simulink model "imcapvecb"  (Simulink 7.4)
settings: Solver=ode45  StartTime=0  StopTime=2.5  MaxStep=5e-4  RelTol=1e-4

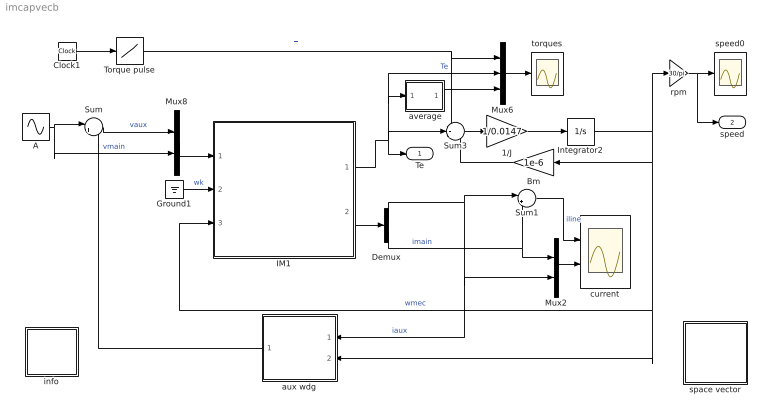
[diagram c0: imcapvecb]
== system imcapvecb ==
  " average" : Subsystem
  1/J : Gain  Gain=1/0.0147  ParameterDataType=sfix(16)  ParameterScaling=2^0  OutDataType=sfix(16)  OutScaling=2^0
  A : Sin  Amplitude=110*sqrt(2)  Bias=0  Frequency=2*pi*60  Phase=pi/2  Samples=10  SampleTime=0
  Bm : Gain  Gain=1e-6  ParameterDataType=sfix(16)  ParameterScaling=2^0  OutDataType=sfix(16)  OutScaling=2^0
  Clock1 : Clock
  Demux : Demux  Outputs=2
  Ground1 : Ground
  IM1 : Subsystem  mask(Inductionmachine){Rs=2.02, Rr=4.12, Lsl=8.54e-3, Lrl=3.13e-3, Lm=180e-3, wo=2*pi*60, p=4}
      mask prompts: Rs "Stator resistance [ohm]"; Rr "Rotor resistance [ohm]"; Lsl "Stator leakage inductance  [H]"; Lrl "Rotor leakage inductance [H]"; Lm "Magnetizing inductance [H]"; wo "Base frequency [rad/s]"; p "Number of poles"
      mask help: Space vector model of the induction machine in a general frame k. SI units
  Integrator2 : Integrator
  Mux2 : Mux  Inputs=2
  Mux6 : Mux  Inputs=3
  Mux8 : Mux  Inputs=2
  Sum : Sum  Inputs=|+-  OutDataType=sfix(16)  OutScaling=2^0
  Sum1 : Sum  Inputs=|++  OutDataType=sfix(16)  OutScaling=2^0
  Sum3 : Sum  Inputs=-+-  OutDataType=sfix(16)  OutScaling=2^0
  Torque pulse : Lookup  InputValues=[0 1 1 1.5 1.5 2]  Table=[0 0 3 3 1.3 1.3]  OutDataType=sfix(16)  OutScaling=2^0
  aux wdg : Subsystem  mask{Cstart=183e-6, p=4, Nsw=3/4}
      mask prompts: Cstart "Start capacitance [F]"; p "Number of poles"; Nsw "Speed when switch disconnects [pu]"
  current : Scope  NumInputPorts=2
  info : Subsystem
  rpm : Gain  Gain=30/pi  ParameterDataType=sfix(16)  ParameterScaling=2^0  OutDataType=sfix(16)  OutScaling=2^0
  space vector : Subsystem
  speed0 : Scope
  torques : Scope
  Te : Outport
  speed : Outport  Port=2
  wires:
  Sum1/1 -> current/1  "iline"
  Mux2/1 -> current/2
  Mux8/1 -> IM1/1(vs)
  Sum/1 -> Mux8/1  "vaux"
  A/1 -> Sum/1, Mux8/2  "vmain"
  IM1/2(is) -> Demux/1
  Demux/1 -> Sum1/1, aux wdg/1(ias), Mux2/2  "iaux"
  Demux/2 -> Sum1/2, Mux2/1  "imain"
  1/J/1 -> Integrator2/1
  Mux6/1 -> torques/1
  Bm/1 -> Sum3/3
  Integrator2/1 -> Bm/1, aux wdg/2(wmec), IM1/3(wmec), rpm/1  "wmec"
  rpm/1 -> speed/1, speed0/1
  IM1/1(Te) -> Sum3/2, Te/1, Mux6/2, " average"/1(sig)  "Te"
  aux wdg/1(vaux) -> Sum/2
  Sum3/1 -> 1/J/1
  Clock1/1 -> Torque pulse/1
  Torque pulse/1 -> Mux6/1, Sum3/1  "Tl"
  Ground1/1 -> IM1/2(wk)  "wk"
  " average"/1(ave) -> Mux6/3

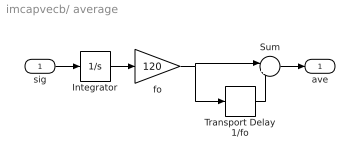
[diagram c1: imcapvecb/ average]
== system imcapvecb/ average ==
  sig : Inport  OutDataType=sfix(16)  OutScaling=2^0
  Integrator : Integrator
  Sum : Sum  Inputs=|+-  OutDataType=sfix(16)  OutScaling=2^0
  Transport Delay 1/fo : TransportDelay  DelayTime=1/120
  fo : Gain  Gain=120  ParameterDataType=sfix(16)  ParameterScaling=2^0  OutDataType=sfix(16)  OutScaling=2^0
  ave : Outport
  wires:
  Sum/1 -> ave/1
  Transport Delay 1/fo/1 -> Sum/2
  sig/1 -> Integrator/1
  fo/1 -> Transport Delay 1/fo/1, Sum/1
  Integrator/1 -> fo/1

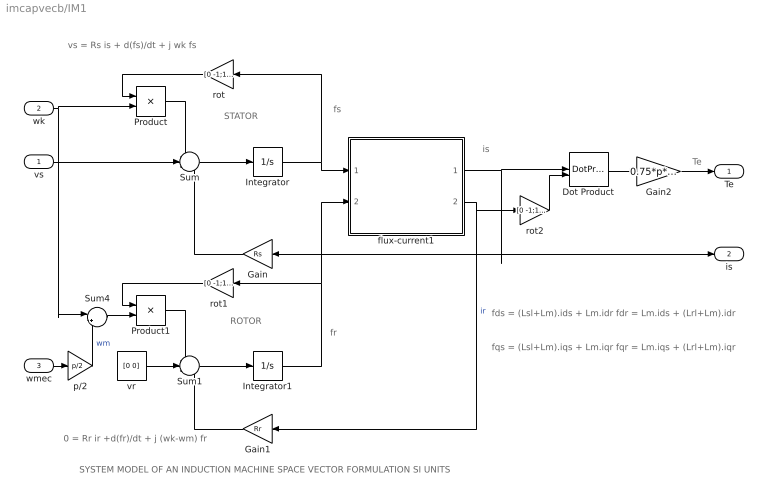
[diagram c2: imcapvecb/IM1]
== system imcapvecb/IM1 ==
  note: ROTOR
  note: STATOR
  note: fs
  note: is
  note: Te
  note: SYSTEM MODEL OF AN INDUCTION MACHINE SPACE VECTOR FORMULATION SI UNITS
  note: vs = Rs is + d(fs)/dt + j wk fs
  note: 0 = Rr ir +d(fr)/dt + j (wk-wm) fr
  note: fds = (Lsl+Lm).ids + Lm.idr fdr = Lm.ids + (Lrl+Lm).idr
  note: fqs = (Lsl+Lm).iqs + Lm.iqr fqr = Lm.iqs + (Lrl+Lm).iqr
  note: fr
  vs : Inport  OutDataType=sfix(16)  OutScaling=2^0
  wk : Inport  Port=2  OutDataType=sfix(16)  OutScaling=2^0
  wmec : Inport  Port=3  OutDataType=sfix(16)  OutScaling=2^0
  Dot Product : DotProduct  OutDataType=fixdt(1, 16)  OutScaling=2^-10
  Gain : Gain  Gain=Rs  ParameterDataType=sfix(16)  ParameterScaling=2^0  OutDataType=sfix(16)  OutScaling=2^0
  Gain1 : Gain  Gain=Rr  ParameterDataType=sfix(16)  ParameterScaling=2^0  OutDataType=sfix(16)  OutScaling=2^0
  Gain2 : Gain  Gain=0.75*p*Lm  ParameterDataType=sfix(16)  ParameterScaling=2^0  OutDataType=sfix(16)  OutScaling=2^0
  Integrator : Integrator  InitialCondition=[0 0]
  Integrator1 : Integrator  InitialCondition=[0 0]
  Product : Product  OutDataType=sfix(16)  OutScaling=2^0
  Product1 : Product  OutDataType=sfix(16)  OutScaling=2^0
  Sum : Sum  Inputs=-+-  OutDataType=sfix(16)  OutScaling=2^0
  Sum1 : Sum  Inputs=-+-  OutDataType=sfix(16)  OutScaling=2^0
  Sum4 : Sum  Inputs=|+-  OutDataType=sfix(16)  OutScaling=2^0
  flux-current1 : Subsystem
  p/2 : Gain  Gain=p/2  ParameterDataType=sfix(16)  ParameterScaling=2^0  OutDataType=sfix(16)  OutScaling=2^0
  rot : Gain  Gain=[0 -1;1 0]  Multiplication=Matrix(K*u)  ParameterDataType=sfix(16)  ParameterScaling=2^0  OutDataType=sfix(16)  OutScaling=2^0
  rot1 : Gain  Gain=[0 -1;1 0]  Multiplication=Matrix(K*u)  ParameterDataType=sfix(16)  ParameterScaling=2^0  OutDataType=sfix(16)  OutScaling=2^0
  rot2 : Gain  Gain=[0 -1;1 0]  Multiplication=Matrix(K*u)  ParameterDataType=sfix(16)  ParameterScaling=2^0  OutDataType=sfix(16)  OutScaling=2^0
  vr : Constant  Value=[0 0]  OutDataType=sfix(16)  OutScaling=2^0
  Te : Outport
  is : Outport  Port=2
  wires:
  Gain/1 -> Sum/3
  vr/1 -> Sum1/2
  Gain1/1 -> Sum1/3
  Integrator/1 -> flux-current1/1(fs), rot/1
  Integrator1/1 -> rot1/1, flux-current1/2(fr)
  Product1/1 -> Sum1/1
  rot1/1 -> Product1/1
  Product/1 -> Sum/1
  rot/1 -> Product/1
  Sum4/1 -> Product1/2
  vs/1 -> Sum/2
  wk/1 -> Product/2, Sum4/1
  Sum1/1 -> Integrator1/1
  Sum/1 -> Integrator/1
  flux-current1/1(is) -> Gain/1, is/1, Dot Product/1
  Dot Product/1 -> Gain2/1
  Gain2/1 -> Te/1
  wmec/1 -> p/2/1
  p/2/1 -> Sum4/2  "wm"
  rot2/1 -> Dot Product/2
  flux-current1/2(ir) -> Gain1/1, rot2/1  "ir"

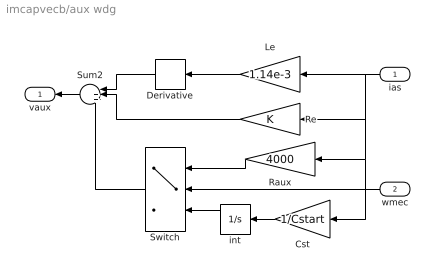
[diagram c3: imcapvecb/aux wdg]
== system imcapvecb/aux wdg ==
  ias : Inport  OutDataType=sfix(16)  OutScaling=2^0
  wmec : Inport  Port=2  OutDataType=sfix(16)  OutScaling=2^0
  Cst : Gain  Gain=1/Cstart  ParameterDataType=sfix(16)  ParameterScaling=2^0  OutDataType=sfix(16)  OutScaling=2^0
  Derivative : Derivative
  Le : Gain  Gain=1.14e-3  ParameterDataType=sfix(16)  ParameterScaling=2^0  OutDataType=sfix(16)  OutScaling=2^0
  Raux : Gain  Gain=4000  ParameterDataType=sfix(16)  ParameterScaling=2^0  OutDataType=sfix(16)  OutScaling=2^0
  Re : Gain  ParameterDataType=sfix(16)  ParameterScaling=2^0  OutDataType=sfix(16)  OutScaling=2^0
  Sum2 : Sum  Inputs=|+++  OutDataType=sfix(16)  OutScaling=2^0
  Switch : Switch  Threshold=Nsw*377*2/p
  int : Integrator
  vaux : Outport
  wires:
  Le/1 -> Derivative/1
  Derivative/1 -> Sum2/1
  Re/1 -> Sum2/2
  Cst/1 -> int/1
  Raux/1 -> Switch/1
  Switch/1 -> Sum2/3
  Sum2/1 -> vaux/1
  wmec/1 -> Switch/2
  ias/1 -> Cst/1, Raux/1, Re/1, Le/1
  int/1 -> Switch/3

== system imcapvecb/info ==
  note: This demo simulates the starting characteristics of a capacitor-start single-phase induction motor

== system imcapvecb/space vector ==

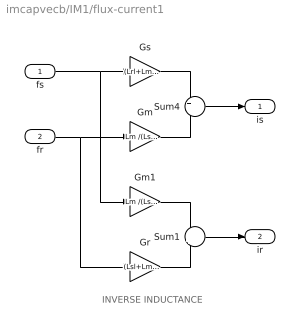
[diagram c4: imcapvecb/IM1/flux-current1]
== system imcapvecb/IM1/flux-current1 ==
  note: INVERSE INDUCTANCE
  fs : Inport  OutDataType=sfix(16)  OutScaling=2^0
  fr : Inport  Port=2  OutDataType=sfix(16)  OutScaling=2^0
  Gm : Gain  Gain=Lm /(Lsl*Lrl+Lsl*Lm+Lrl*Lm)  ParameterDataType=sfix(16)  ParameterScaling=2^0  OutDataType=sfix(16)  OutScaling=2^0
  Gm1 : Gain  Gain=Lm /(Lsl*Lrl+Lsl*Lm+Lrl*Lm)  ParameterDataType=sfix(16)  ParameterScaling=2^0  OutDataType=sfix(16)  OutScaling=2^0
  Gr : Gain  Gain=(Lsl+Lm )/(Lsl*Lrl+Lsl*Lm+Lrl*Lm)  ParameterDataType=sfix(16)  ParameterScaling=2^0  OutDataType=sfix(16)  OutScaling=2^0
  Gs : Gain  Gain=(Lrl+Lm) /(Lsl*Lrl+Lsl*Lm+Lrl*Lm)  ParameterDataType=sfix(16)  ParameterScaling=2^0  OutDataType=sfix(16)  OutScaling=2^0
  Sum1 : Sum  Inputs=-+  OutDataType=sfix(16)  OutScaling=2^0
  Sum4 : Sum  Inputs=+-  OutDataType=sfix(16)  OutScaling=2^0
  is : Outport
  ir : Outport  Port=2
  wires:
  fs/1 -> Gs/1, Gm1/1
  Gs/1 -> Sum4/1
  fr/1 -> Gm/1, Gr/1
  Gm/1 -> Sum4/2
  Sum4/1 -> is/1
  Gm1/1 -> Sum1/1
  Gr/1 -> Sum1/2
  Sum1/1 -> ir/1
